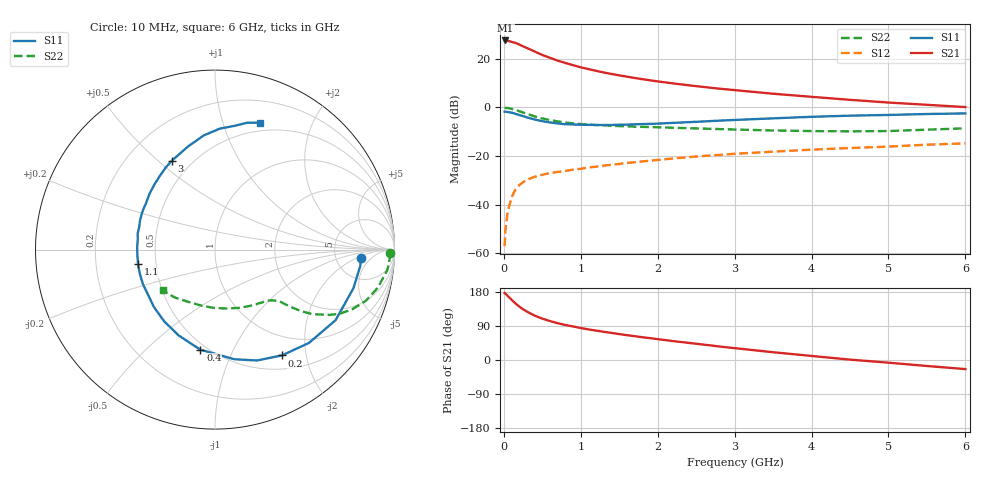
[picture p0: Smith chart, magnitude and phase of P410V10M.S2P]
! SIEMENS Small Signal Semiconductors
! BFP182
! Si NPN RF Bipolar Junction Transistor in SOT143
! VCE = 10 V  IC = 10 mA
! Common Emitter S-Parameters:  March  1996
# GHz  S  MA  R  50
!  f  S11  S21  S12  S22
! GHz  MAG  ANG  MAG  ANG  MAG  ANG  MAG  ANG
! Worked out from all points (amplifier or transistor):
!   36 points, 10 MHz to 6 GHz, reference 50 ohm
!   highest |S21| = 27.5 dB at 20 MHz (marker M1)
!   |S21| within 3 dB of that: start of sweep to 293.1 MHz
!   unconditionally stable (mu >= 1): 1.306 GHz to 5.763 GHz
!   at 250 MHz: K = 0.31, MSG = 27.9 dB, |S12| = -30.8 dB
!   at 1.4 GHz: K = 1.03, MAG = 17.6 dB, |S12| = -23.6 dB
!   at 6 GHz: K = 0.98, MSG = 7.5 dB, |S12| = -14.8 dB
!   S11 on the Smith chart (normalised r, x): 10 MHz: 9.13, -2.39; 200 MHz: 0.69, -1.59; 400 MHz: 0.46, -0.75; 1.1 GHz: 0.39, -0.08; 3 GHz: 0.39, +0.56; 6 GHz: 0.41, +1.34
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0.01  0.8142 -3.1  23.53 177.0  0.0014 82.4  0.9773 -1.2
0.02  0.8147 -6.4  23.72 175.5  0.003 78.5  0.9754 -2.7
0.05  0.8007 -15.6  23.45 168.9  0.0071 82.0  0.9666 -6.8
0.1  0.7785 -30.3  22.14 159.1  0.0141 73.9  0.9314 -13.2
0.15  0.7379 -44.8  21.11 149.5  0.0203 68.1  0.8871 -18.8
0.2  0.6974 -57.7  19.64 141.1  0.0251 62.0  0.8349 -23.4
0.25  0.6605 -69.3  17.94 133.9  0.0289 58.0  0.7846 -27.0
0.3  0.6203 -80.0  16.62 127.8  0.0326 54.7  0.7348 -29.7
0.4  0.5636 -98.3  14.07 117.1  0.0373 49.7  0.6515 -33.5
0.5  0.5193 -113.0  11.91 109.2  0.0411 46.9  0.591 -35.5
0.6  0.4896 -125.4  10.43 102.7  0.0446 45.6  0.5477 -36.6
0.7  0.4669 -136.8  9.109 97.2  0.047 44.5  0.5144 -37.5
0.9  0.445 -154.8  7.363 88.5  0.0523 43.9  0.4684 -38.5
1.1  0.4369 -169.2  6.116 80.7  0.058 43.5  0.4429 -40.0
1.3  0.4339 178.5  5.202 74.4  0.0634 43.3  0.4256 -41.6
1.6  0.4407 163.3  4.275 65.6  0.0717 43.1  0.4067 -44.8
2.2  0.4793 139.6  3.106 49.9  0.0889 41.2  0.3807 -53.1
3  0.5507 115.9  2.262 31.3  0.1109 36.0  0.3506 -67.9
3.5  0.5941 104.6  1.906 20.5  0.1227 32.1  0.3345 -78.8
4.5  0.6747 87.7  1.428 1.0  0.1459 24.6  0.3211 -103.8
5.5  0.7297 75.7  1.128 -15.8  0.1709 17.9  0.3477 -129.6
6  0.7509 70.3  1.013 -24.0  0.1815 13.4  0.3701 -142.0
